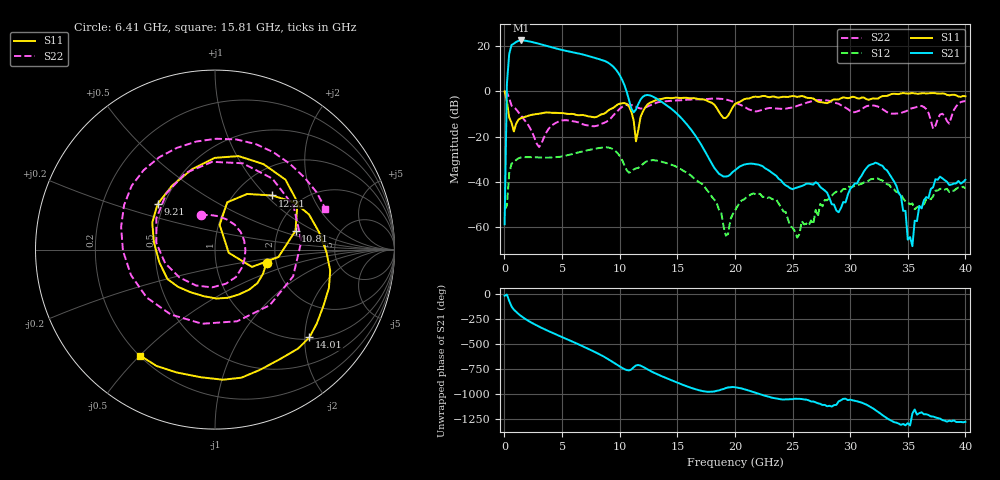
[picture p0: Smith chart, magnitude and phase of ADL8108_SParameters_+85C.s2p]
! Analog Devices, Inc.
! Device:	ADL8108 SN8565
! Description:	"GaAs, pHEMT, MMIC, Low Noise Amplifier, 1.5 GHz to 6 GHz"
! Conditions:	Vdd = 5.0 V
!		Idq = 90 mA
!  Rbias = 1270 Ohm
!		Pin = -25 dBm
!		Operating Temperature = +85 C (at package bottom)
! Board loss de-embedded from S21 magnitude.  All other RF measurements reference to RF coaxial connector.
! Frequency (GHz)	S11_Mag (dB)	S11_Phase (deg)	S21_Mag (dB)	S21_Phase (deg)	S12_Mag (dB)	S12_Phase (deg)	S22_Mag (dB)	S22_Phase (deg)
#  GHZ  S  DB  R 50
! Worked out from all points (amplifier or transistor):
!   201 points, 10 MHz to 40 GHz, reference 50 ohm
!   highest |S21| = 22.6 dB at 1.41 GHz (marker M1)
!   |S21| within 3 dB of that: 560.7 MHz to 4.08 GHz (3.519 GHz wide, 152 % of centre)
!   unconditionally stable (mu >= 1): 206 MHz to end of sweep
!   at 6.61 GHz: K = 1.51, MAG = 17.5 dB, |S12| = -26.8 dB
!   at 20 GHz: K = 6036.60, MAG = -31.9 dB, |S12| = -52.9 dB
!   at 40 GHz: K = 1543.56, MAG = -33.0 dB, |S12| = -42.9 dB
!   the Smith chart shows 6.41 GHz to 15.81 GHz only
!   S11 on the Smith chart (normalised r, x): 6.41 GHz: 1.78, -0.28; 9.21 GHz: 0.46, +0.28; 10.81 GHz: 2.50, +0.67; 12.21 GHz: 1.46, +1.09; 14.01 GHz: 1.04, -2.11; 15.81 GHz: 0.20, -0.50
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0.01  0.01 -5.3  -58.87 -13.5  -52.29 -177.5  -0.01 -2.3
0.21  -4.51 -96.6  3.34 -2.2  -50.66 178.5  -0.43 -49.0
0.41  -11.52 -128.5  16.66 -66.2  -36.19 126.6  -2.97 -95.3
0.61  -13.83 -145.2  20.56 -121.0  -32.02 79.4  -6.28 -118.0
1.01  -14.32 -133.4  21.92 -175.7  -30.36 36.7  -7.90 -162.4
1.41  -11.87 -158.5  22.60 144.7  -29.29 7.3  -10.53 157.7
2.21  -10.53 164.9  22.12 84.4  -29.14 -30.7  -16.14 92.4
3.41  -9.41 121.2  20.54 12.8  -29.33 -70.6  -20.55 -79.0
4.81  -9.57 67.7  18.61 -59.8  -28.95 -108.0  -13.10 -162.4
6.41  -10.56 -14.1  16.85 -141.1  -27.02 -155.2  -13.69 113.0
6.81  -10.42 -38.2  16.37 -162.4  -26.54 -169.8  -14.56 84.7
8.21  -10.68 -134.8  14.33 120.0  -25.05 133.8  -14.87 -34.8
9.21  -7.78 141.6  11.97 53.9  -25.12 79.9  -11.98 -142.0
10.81  -6.73 13.2  -3.84 -43.7  -36.06 31.9  -5.87 51.1
12.21  -7.14 43.3  -1.71 -20.0  -31.37 19.3  -7.18 -124.2
13.41  -3.48 -18.6  -3.81 -89.9  -30.92 -38.5  -4.66 142.6
14.01  -2.87 -42.9  -5.94 -119.0  -31.66 -63.1  -4.36 110.6
15.81  -2.82 -125.2  -14.48 157.3  -35.96 -139.0  -3.66 20.4
20.2  -5.01 155.5  -34.12 143.3  -51.05 -164.4  -5.35 -171.6
26.8  -3.13 -81.6  -41.26 5.0  -58.80 111.8  -4.21 116.0
33.4  -1.57 111.8  -36.63 -177.5  -41.44 -116.8  -9.60 122.1
40  -2.15 -7.4  -39.13 160.6  -42.92 148.5  -4.26 -31.9
